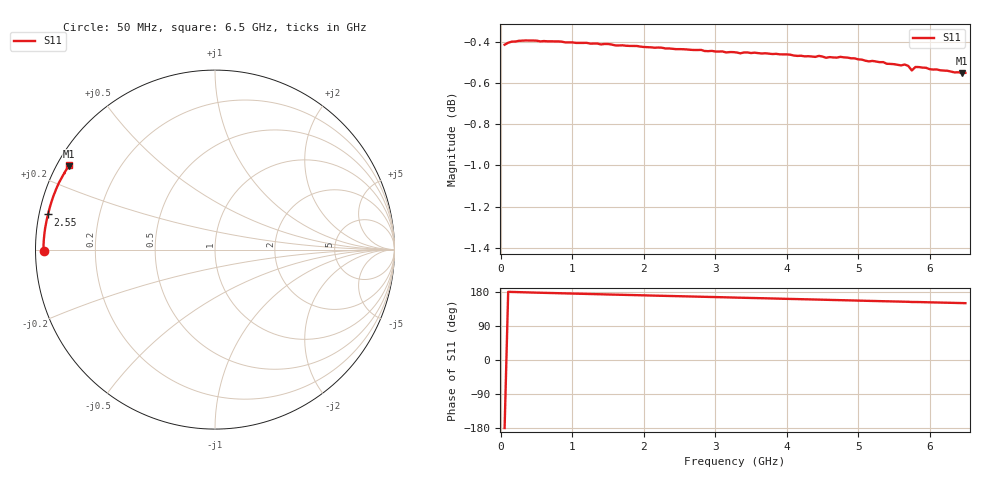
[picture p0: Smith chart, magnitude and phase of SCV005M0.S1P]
! Infineon Technologies  Discrete & RF Semiconductors
! BAR63-02L
! Si PIN Diode in TSLP-2
! IF = 5 mA
! S-Parameters:  March  2002
# GHz  S  MA  R  50
!  f  S11
! GHz  MAG  ANG
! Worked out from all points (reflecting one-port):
!   130 points, 50 MHz to 6.5 GHz, reference 50 ohm
!   lowest |S11| = -0.6 dB at 6.45 GHz (marker M1), VSWR 31.53, Z = 1.7 + j13.3 ohm
!   phase of S11 starts at -180 deg and turns -30 deg over the sweep
!   S11 on the Smith chart (normalised r, x): 50 MHz: 0.02, -0.00; 2.55 GHz: 0.03, +0.10; 6.5 GHz: 0.03, +0.27
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0.05  0.9535 -179.5
0.1  0.9546 179.9
0.3  0.9557 178.7
0.7  0.9554 176.7
0.9  0.9548 175.8
1.2  0.9545 174.3
1.7  0.9532 172.0
2.5  0.9512 168.3
2.55  0.9511 168.1
2.6  0.951 167.8
2.75  0.9507 167.2
2.8  0.9508 166.9
3.1  0.9499 165.6
3.3  0.9494 164.6
3.6  0.949 163.2
3.75  0.9488 162.6
4.1  0.9477 160.9
4.25  0.9473 160.3
4.9  0.9463 157.2
5.3  0.9443 155.4
5.35  0.9443 155.1
5.7  0.9423 153.6
5.75  0.9399 153.1
5.8  0.9417 153.1
5.85  0.9417 152.9
5.9  0.9414 152.6
6.45  0.9385 150.2
6.5  0.9386 150.0
